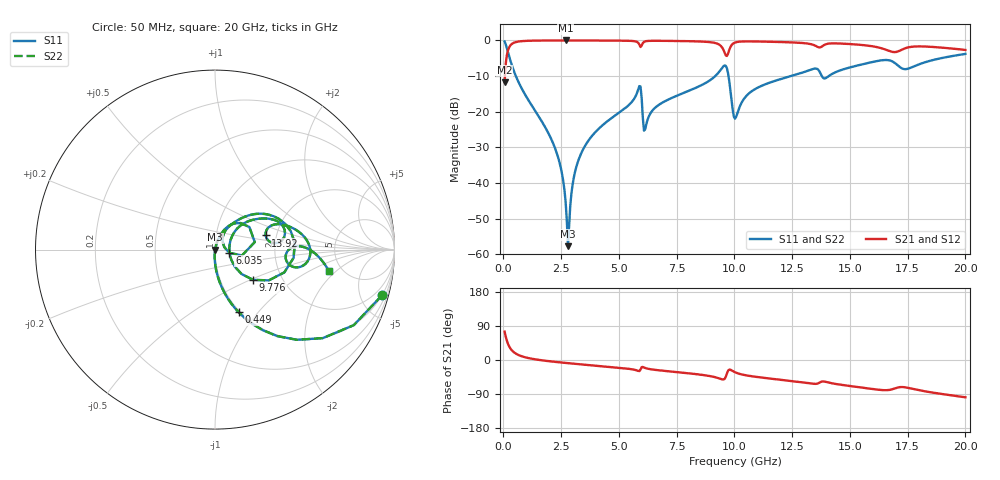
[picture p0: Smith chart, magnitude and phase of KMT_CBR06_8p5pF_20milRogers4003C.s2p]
! Data measured by Modelithics Inc. support@modelithics.com 813-866-6335
! KEMET CBR0603 8.5pF, Pad Width= 0.851mm, Pad Length= 0.64mm, Pad Gap= 0.62mm, 20mil Rogers 4003C substrate Data, January 2022
# hz S ma R 50
! 2 Port Network Data from SP1.SP block
! freq  magS11  angS11  magS21  angS21  magS12  angS12  magS22  angS22
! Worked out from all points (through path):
!   401 points, 50 MHz to 20 GHz, reference 50 ohm
!   highest |S21| = -0.01 dB at 2.693 GHz (marker M1); lowest = -11.7 dB at 50 MHz (marker M2)
!   group delay of S21, straight-line fit = 14.5 ps
!   lowest |S11| = -57.7 dB at 2.793 GHz (marker M3), VSWR 1.00, Z = 50.1 - j0.0381 ohm
!   |S11| at or under -10 dB: 537.3 MHz to 9.169 GHz (8.632 GHz wide, 178 % of centre); 9.744 GHz to 12.44 GHz (2.701 GHz wide, 24.3 % of centre); 13.79 GHz to 14.09 GHz (300.1 MHz wide, 2.15 % of centre)
!   |S22| runs from -57.7 to -0.3 dB; largest |S21 - S12| = 0
!   S11 on the Smith chart (normalised r, x): 50 MHz: 0.98, -7.36; 449 MHz: 0.98, -0.80; 6.035 GHz: 1.17, -0.04; 9.776 GHz: 1.43, -0.52; 13.92 GHz: 1.75, +0.30; 20 GHz: 3.94, -1.64
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5e7  0.9655 -15.2  0.2599 74.8  0.2599 74.8  0.9655 -15.2
4.49e8  0.3739 -69.3  0.9266 20.6  0.9266 20.6  0.3739 -69.3
2.194625e9  0.03321 -92.7  0.9982 -4.7  0.9982 -4.7  0.03321 -92.7
2.54375e9  0.01305 -91.4  0.9986 -6.9  0.9986 -6.9  0.01305 -91.4
2.693375e9  0.005337 -84.0  0.9986 -7.7  0.9986 -7.7  0.005337 -84.0
2.793125e9  0.001302 -17.0  0.9986 -8.3  0.9986 -8.3  0.001302 -17.0
3.092375e9  0.01402 74.4  0.9984 -10.0  0.9984 -10.0  0.01402 74.4
3.391625e9  0.02723 75.3  0.9981 -11.7  0.9981 -11.7  0.02723 75.3
5.8355e9  0.2055 46.0  0.9259 -28.8  0.9259 -28.8  0.2055 46.0
6.035e9  0.08178 -12.6  0.9184 -18.4  0.9184 -18.4  0.08178 -12.6
6.184625e9  0.06664 50.8  0.9781 -22.0  0.9781 -22.0  0.06664 50.8
6.73325e9  0.1253 60.8  0.9875 -27.2  0.9875 -27.2  0.1253 60.8
9.276875e9  0.3435 35.2  0.8955 -47.4  0.8955 -47.4  0.3435 35.2
9.576125e9  0.4461 4.9  0.6726 -49.6  0.6726 -49.6  0.4461 4.9
9.775625e9  0.271 -38.5  0.7338 -25.4  0.7338 -25.4  0.271 -38.5
1.0025e10  0.07989 2.3  0.9328 -32.2  0.9328 -32.2  0.07989 2.3
1.087288e10  0.2057 42.9  0.9669 -43.9  0.9669 -43.9  0.2057 42.9
1.336662e10  0.3943 21.5  0.877 -62.4  0.877 -62.4  0.3943 21.5
1.391525e10  0.2929 15.6  0.8723 -57.1  0.8723 -57.1  0.2929 15.6
1.670825e10  0.5251 -5.9  0.7108 -79.0  0.7108 -79.0  0.5251 -5.9
1.74065e10  0.3955 -4.8  0.7783 -72.2  0.7783 -72.2  0.3955 -4.8
2e10  0.6467 -10.8  0.7351 -98.4  0.7351 -98.4  0.6467 -10.8
